FUNCTION_BLOCK FB_IEDGse IMPLEMENTS I_GseLinkStatusEventSink
VAR_INPUT
	fbAdapter		: FB_GseAdapterClass := (ipLinkStatus:=THIS^);
END_VAR
VAR
	eLinkStatus		: E_GseLinkStatus;
	
	bSuccess		: BOOL;
	ipError			: I_ServiceErrorClass;
	
	bSubscribe		: BOOL := TRUE; (* Rising edge enables subscriber GoCB's *)
	bUnsubscribe	: BOOL; (* Rising edge disables subscriber GoCB's *)
END_VAR

(*=========================================================================================*)
bSuccess:= fbAdapter.Execute(ipError=>ipError); (* Execute network adapter *)

(*=========================================================================================*)
IF bSubscribe THEN (* Enable subscriber GoCB's *)
	bSubscribe:= FALSE;
	bSuccess:= fbIED.IEDLD1.LLN0.gocb01.Subscriber.Enable(ipAdapter:=fbAdapter, ipError=>ipError);
	bSuccess:= fbIED.IEDLD1.LLN0.gocb02.Subscriber.Enable(ipAdapter:=fbAdapter, ipError=>ipError);
	bSuccess:= fbIED.IEDLD1.LLN0.gocb03.Subscriber.Enable(ipAdapter:=fbAdapter, ipError=>ipError);
ELSIF bUnsubscribe THEN (* Disable subscriber GoCB's *)
	bUnsubscribe:= FALSE;
	bSuccess:= fbIED.IEDLD1.LLN0.gocb01.Subscriber.Disable(ipError=>ipError);
	bSuccess:= fbIED.IEDLD1.LLN0.gocb02.Subscriber.Disable(ipError=>ipError);
	bSuccess:= fbIED.IEDLD1.LLN0.gocb03.Subscriber.Disable(ipError=>ipError);
ELSE (* Execute subscriber GoCB's *)
	bSuccess:= fbIED.IEDLD1.LLN0.gocb01.Subscriber.Execute(ipError=>ipError);
	bSuccess:= fbIED.IEDLD1.LLN0.gocb02.Subscriber.Execute(ipError=>ipError);
	bSuccess:= fbIED.IEDLD1.LLN0.gocb03.Subscriber.Execute(ipError=>ipError);
END_IF

(* This method is called every time the network adapter link status changes. *)
METHOD OnLinkStatusChange
VAR_INPUT
	ipAdapter	: I_GseAdapterClass;
	eStatus		: E_GseLinkStatus;
END_VAR
VAR
END_VAR
eLinkStatus:= eStatus;
END_METHOD

END_FUNCTION_BLOCK
